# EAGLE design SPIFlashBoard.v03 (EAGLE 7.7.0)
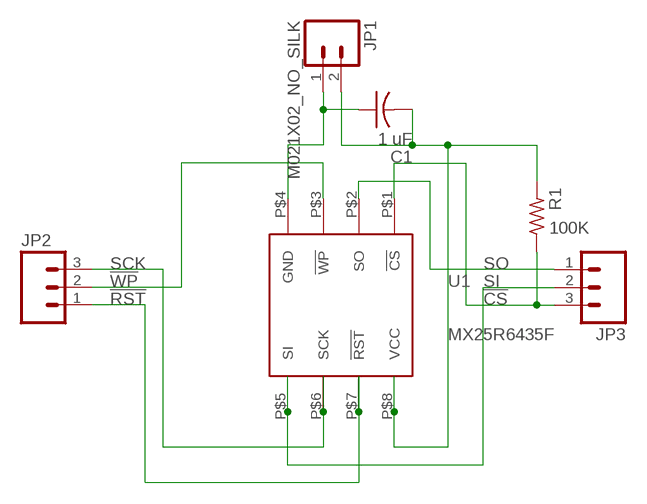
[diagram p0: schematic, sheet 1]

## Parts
C1  1 uF  C-US  [C0402_B]
JP1  M021X02_NO_SILK  [1X02_NO_SILK]
JP2  M031X03_NO_SILK  [1X03_NO_SILK]
JP3  M031X03_NO_SILK  [1X03_NO_SILK]
R1  100K  R-US_  [R0402_B]
U1  MX25R6435F  [MX25R6435F]

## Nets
!CS: JP3.3 R1.1 U1.P$1(!CS)
!RST: JP2.1 U1.P$7(!RST)
!WP: JP2.2 U1.P$3(!WP)
GND: C1.1 JP1.1 U1.P$4(GND)
N$3: C1.2 JP1.2 R1.2 U1.P$8(VCC)
SCK: JP2.3 U1.P$6(SCK)
SI: JP3.2 U1.P$5(SI)
SO: JP3.1 U1.P$2(SO)

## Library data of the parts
C1 = Spark:C-US: Capacitor
JP1 = SparkFun-Connectors:M02: Standard 2-pin 0.1" header. Use with
JP2 JP3 = SparkFun-Connectors:M03: Header 3 Standard 3-pin 0.1" header. Use with straight break away headers (SKU : PRT-00116), right angle break away headers (PRT-00553), swiss pins (PRT-00743), machine pins (PRT-00117), and female headers (PRT-00115). Molex polarized connector foot print use with SKU : PRT-08232 with associated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
R1 = Spark:R-US_: 0402 Resistor
U1 = Kris:MX25R6435F: MX25R6435F 64 MBit SPI NOR Flash from Macronix

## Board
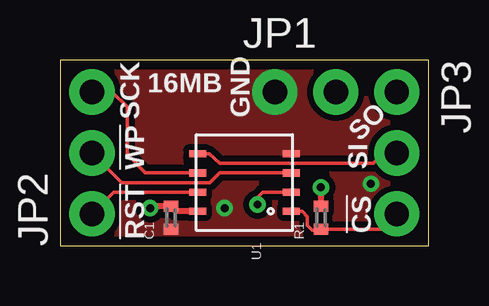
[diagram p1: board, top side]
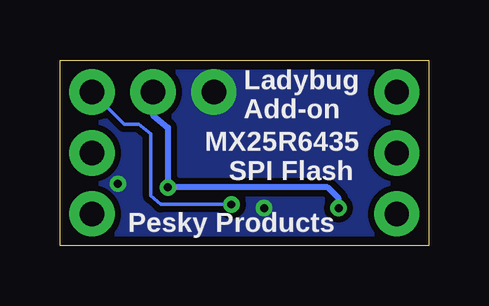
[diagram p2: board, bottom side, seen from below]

Size 15.37 x 7.75 mm. Coordinates in mm from the lower left corner, seen from the top.
Outline: 0,0 15.37,0 15.37,7.75 0,7.75 0,0
Copper layers (1*16): Top 0.0356mm / dielectric 1.5011mm / Bottom 0.0356mm
Design rules "oshpark-2layer *": minimum track width 6mil, minimum drill 13mil, track to track 6mil, track to pad 6mil, pad to pad 6mil, via to via 6mil, smd to smd 6mil, copper to edge 15mil, drill to drill 6mil, minimum pad ring 7mil, minimum via ring 7mil, stop-mask expansion 4mil, vias tented up to drill 20mil, thermal gap 10mil

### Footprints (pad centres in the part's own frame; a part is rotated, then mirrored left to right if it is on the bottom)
C0402_B = smd 0.457 x 0.61: 1 -0.483,0; 2 0.483,0
1X02_NO_SILK = drill 1.016 pad 1.88: 1 0,0; 2 2.54,0
1X03_NO_SILK = drill 1.016 pad 1.88: 1 0,0; 2 2.54,0; 3 5.08,0
R0402_B = smd 0.457 x 0.61: 1 -0.483,0; 2 0.483,0
MX25R6435F = smd 0.3 x 0.7: P$1 1.2,1.95; P$2 0.4,1.95; P$3 -0.4,1.95; P$4 -1.2,1.95; P$5 -1.2,-1.95; P$6 -0.4,-1.95; P$7 0.4,-1.95; P$8 1.2,-1.95

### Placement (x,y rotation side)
C1  4.62,1.17 90 top
JP1  8.95,6.41 0 top
JP2  1.33,1.33 90 top
JP3  14.03,6.41 270 top
R1  10.87,1.17 90 top
U1  7.68,2.64 270 top

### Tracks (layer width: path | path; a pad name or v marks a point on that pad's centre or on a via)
!CS
  Top 0.152: U1.P$1 10.09,1.44 10.31,1.22 10.31,0.86 10.52,0.66 11.05,0.66 R1.1 13.39,0.69 JP3.3
!RST
  Top 0.152: U1.P$7 2.24,2.24 JP2.1
!WP
  Top 0.152: U1.P$3 6.65,3.04 6.25,2.64 2.57,2.64 JP2.2
GND  (via drill 0.33)
  other vias: 6.86,1.57 12.95,2.59
  pour Bottom (isolate 0.254, no thermals): 0,7.75 0,0 15.37,0 15.37,7.75
  pour Top (isolate 0.254, no thermals): 0,7.8 0,0.05 15.37,0 15.37,7.75
N$3  (via drill 0.33)
  Top 0.254: U1.P$8 4.83,1.44 C1.2 3.89,1.65 v3.76,1.57 | v10.87,2.44 R1.2
  Bottom 0.254: JP1.2 11.49,5.45 10.87,4.93 v10.87,2.44 4.22,2.44 3.76,1.98 v3.76,1.57
SCK
  Top 0.152: U1.P$6 3.56,3.04 2.79,3.81 2.79,5.79 2.18,6.4 1.35,6.4 JP2.3
SI
  Top 0.152: U1.P$5 6.22,3.84 6.66,3.45 13.06,3.45 13.46,3.86 JP3.2
SO  (via drill 0.33)
  Top 0.152: U1.P$2 8.44,2.24 8.23,2.03 v8.23,1.73
  Bottom 0.152: v8.23,1.73 11.18,1.73 11.58,2.08 11.58,4.67 12.09,5.08 12.7,5.08 JP3.1

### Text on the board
tPlace: 16MB | SCK | GND | SO | !WP | SI | !CS | !RST
bPlace: Ladybug / Add-on | SPI Flash | MX25R6435 | Pesky Products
